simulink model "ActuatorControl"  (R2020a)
settings: Solver=FixedStepDiscrete  StartTime=0.0  StopTime=10.0  FixedStep=0.001  RelTol=1e-3  EnableMultiTasking=on
model workspace (MAT data in the model file):
  Ts : Simulink.Parameter (value not decoded)
symbols that are objects in the model workspace (value not decoded): Ts
undefined symbols (not defined in the file or in its folder): DiscIntNeverNeededParam
libraries: simulink x3

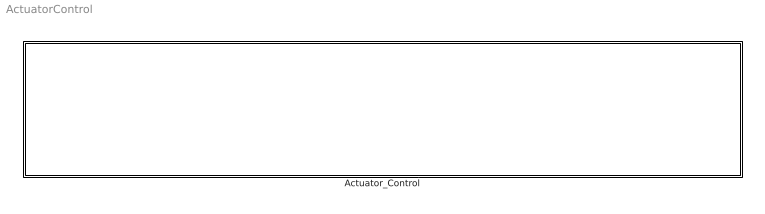
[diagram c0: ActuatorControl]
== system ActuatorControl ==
  Actuator_Control : Subsystem  TreatAsAtomicUnit=on

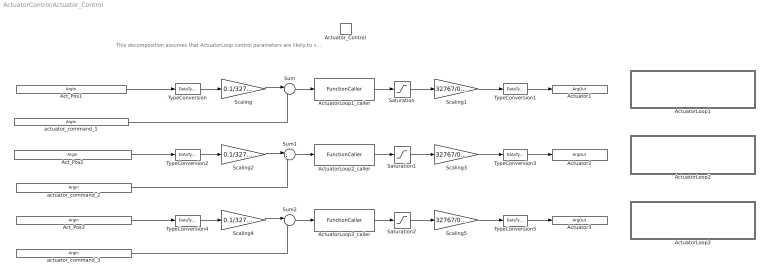
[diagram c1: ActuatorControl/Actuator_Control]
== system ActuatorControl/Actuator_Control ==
  note: This decomposition assumes that ActuatorLoop control parameters are likely to vary between actuators.
  Actuator_Control : TriggerPort  TriggerType=function-call  IsSimulinkFunction=on  FunctionName=Actuator_Control  FunctionVisibility=scoped  VariantControl=Variant  PortDimensions=1
  ActuatorLoop1 : Subsystem  TreatAsAtomicUnit=on
  ActuatorLoop1_caller : FunctionCaller  FunctionPrototype=Y = ActuatorLoop1(U)  InputArgumentSpecifications=double(1)  OutputArgumentSpecifications=double(1)
  ActuatorLoop2 : Subsystem  TreatAsAtomicUnit=on
  ActuatorLoop2_caller : FunctionCaller  FunctionPrototype=Y = ActuatorLoop2(U)  InputArgumentSpecifications=double(1)  OutputArgumentSpecifications=double(1)
  ActuatorLoop3 : Subsystem  TreatAsAtomicUnit=on
  ActuatorLoop3_caller : FunctionCaller  FunctionPrototype=Y = ActuatorLoop3(U)  InputArgumentSpecifications=double(1)  OutputArgumentSpecifications=double(1)
  Saturation : Saturate  UpperLimit=0.3  LowerLimit=-0.3
  Saturation1 : Saturate  UpperLimit=0.3  LowerLimit=-0.3
  Saturation2 : Saturate  UpperLimit=0.3  LowerLimit=-0.3
  Scaling : Gain  Gain=0.1/32767
  Scaling1 : Gain  Gain=32767/0.3  SaturateOnIntegerOverflow=on
  Scaling2 : Gain  Gain=0.1/32767
  Scaling3 : Gain  Gain=32767/0.3  SaturateOnIntegerOverflow=on
  Scaling4 : Gain  Gain=0.1/32767
  Scaling5 : Gain  Gain=32767/0.3  SaturateOnIntegerOverflow=on
  Sum : Sum  Inputs=|-+
  Sum1 : Sum  Inputs=|-+
  Sum2 : Sum  Inputs=|-+
  TypeConversion : DataTypeConversion  OutDataTypeStr=double
  TypeConversion1 : DataTypeConversion  OutDataTypeStr=int16
  TypeConversion2 : DataTypeConversion  OutDataTypeStr=double
  TypeConversion3 : DataTypeConversion  OutDataTypeStr=int16
  TypeConversion4 : DataTypeConversion  OutDataTypeStr=double
  TypeConversion5 : DataTypeConversion  OutDataTypeStr=int16
  Act_Pos1 : ArgIn  OutMin=-32768  OutMax=32767  OutDataTypeStr=int16  ArgumentName=Act_Pos1
  actuator_command_1 : ArgIn  Port=2  OutMin=-.1  OutMax=.1  ArgumentName=actuator_command_1
  Act_Pos2 : ArgIn  Port=3  OutMin=-32768  OutMax=32767  OutDataTypeStr=int16  ArgumentName=Act_Pos2
  actuator_command_2 : ArgIn  Port=4  OutMin=-.1  OutMax=.1  ArgumentName=actuator_command_2
  Act_Pos3 : ArgIn  Port=5  OutMin=-32768  OutMax=32767  OutDataTypeStr=int16  ArgumentName=Act_Pos3
  actuator_command_3 : ArgIn  Port=6  OutMin=-.1  OutMax=.1  ArgumentName=actuator_command_3
  Actuator1 : ArgOut  OutMin=-32768  OutMax=32767  OutDataTypeStr=int16  ArgumentName=Actuator1
  Actuator2 : ArgOut  Port=2  OutMin=-32768  OutMax=32767  OutDataTypeStr=int16  ArgumentName=Actuator2
  Actuator3 : ArgOut  Port=3  OutMin=-32768  OutMax=32767  OutDataTypeStr=int16  ArgumentName=Actuator3
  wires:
  ActuatorLoop1_caller/1 -> Saturation/1
  Saturation/1 -> Scaling1/1
  Scaling/1 -> Sum/1
  Scaling1/1 -> TypeConversion1/1
  Sum/1 -> ActuatorLoop1_caller/1
  actuator_command_1/1 -> Sum/2
  Act_Pos1/1 -> TypeConversion/1
  TypeConversion1/1 -> Actuator1/1
  TypeConversion/1 -> Scaling/1
  Scaling3/1 -> TypeConversion3/1
  TypeConversion2/1 -> Scaling2/1
  Sum1/1 -> ActuatorLoop2_caller/1
  TypeConversion3/1 -> Actuator2/1
  Scaling2/1 -> Sum1/1
  actuator_command_2/1 -> Sum1/2
  Saturation1/1 -> Scaling3/1
  Act_Pos2/1 -> TypeConversion2/1
  ActuatorLoop2_caller/1 -> Saturation1/1
  ActuatorLoop3_caller/1 -> Saturation2/1
  Scaling5/1 -> TypeConversion5/1
  actuator_command_3/1 -> Sum2/2
  Saturation2/1 -> Scaling5/1
  Act_Pos3/1 -> TypeConversion4/1
  Scaling4/1 -> Sum2/1
  TypeConversion5/1 -> Actuator3/1
  Sum2/1 -> ActuatorLoop3_caller/1
  TypeConversion4/1 -> Scaling4/1

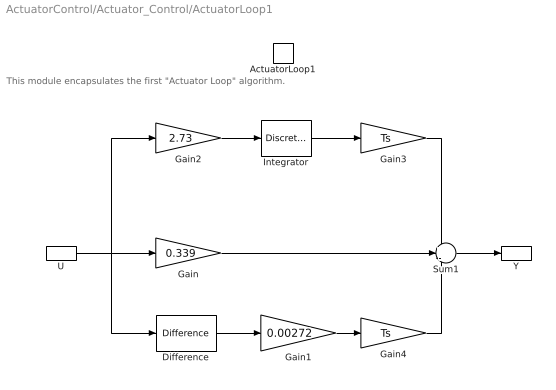
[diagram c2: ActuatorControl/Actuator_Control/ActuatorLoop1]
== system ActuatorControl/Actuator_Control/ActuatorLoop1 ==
  note: This module encapsulates the first "Actuator Loop" algorithm.
  ActuatorLoop1 : TriggerPort  TriggerType=function-call  IsSimulinkFunction=on  FunctionName=ActuatorLoop1  FunctionVisibility=scoped  VariantControl=Variant  PortDimensions=1
  Difference : simulink/Discrete/Difference  ICPrevInput=0.0  OutMin=[]  OutMax=[]  OutDataType=fixdt(1, 16)  OutScaling=2^-10  DoSatur=off
  Gain : Gain  Gain=0.339
  Gain1 : Gain  Gain=0.00272
  Gain2 : Gain  Gain=2.73
  Gain3 : Gain  Gain=Ts
  Gain4 : Gain  Gain=Ts
  Integrator : DiscreteIntegrator  IntegratorMethod=Accumulation: Forward Euler  SampleTime=-1  LimitOutput=on  UpperSaturationLimit=0.1  LowerSaturationLimit=-0.1  ICPrevOutput=DiscIntNeverNeededParam  ICPrevScaledInput=DiscIntNeverNeededParam
  Sum1 : Sum  Inputs=++-
  U : ArgIn  ArgumentName=U
  Y : ArgOut  ArgumentName=Y
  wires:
  Gain1/1 -> Gain4/1
  Sum1/1 -> Y/1
  U/1 -> Difference/1, Gain2/1, Gain/1
  Integrator/1 -> Gain3/1
  Gain2/1 -> Integrator/1
  Gain/1 -> Sum1/2
  Difference/1 -> Gain1/1
  Gain3/1 -> Sum1/1
  Gain4/1 -> Sum1/3

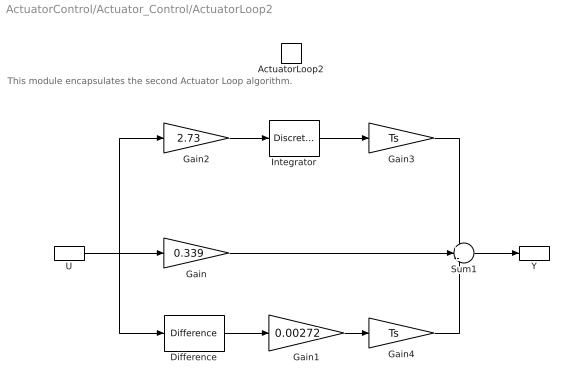
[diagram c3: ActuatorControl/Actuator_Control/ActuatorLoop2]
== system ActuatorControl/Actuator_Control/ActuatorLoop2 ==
  note: This module encapsulates the second Actuator Loop algorithm.
  ActuatorLoop2 : TriggerPort  TriggerType=function-call  IsSimulinkFunction=on  FunctionName=ActuatorLoop2  FunctionVisibility=scoped  VariantControl=Variant  PortDimensions=1
  Difference : simulink/Discrete/Difference  ICPrevInput=0.0  OutMin=[]  OutMax=[]  OutDataType=fixdt(1, 16)  OutScaling=2^-10  DoSatur=off
  Gain : Gain  Gain=0.339
  Gain1 : Gain  Gain=0.00272
  Gain2 : Gain  Gain=2.73
  Gain3 : Gain  Gain=Ts
  Gain4 : Gain  Gain=Ts
  Integrator : DiscreteIntegrator  IntegratorMethod=Accumulation: Forward Euler  SampleTime=-1  LimitOutput=on  UpperSaturationLimit=0.1  LowerSaturationLimit=-0.1  ICPrevOutput=DiscIntNeverNeededParam  ICPrevScaledInput=DiscIntNeverNeededParam
  Sum1 : Sum  Inputs=++-
  U : ArgIn  ArgumentName=U
  Y : ArgOut  ArgumentName=Y
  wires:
  Difference/1 -> Gain1/1
  Gain/1 -> Sum1/2
  Gain2/1 -> Integrator/1
  Integrator/1 -> Gain3/1
  U/1 -> Gain/1, Gain2/1, Difference/1
  Sum1/1 -> Y/1
  Gain1/1 -> Gain4/1
  Gain3/1 -> Sum1/1
  Gain4/1 -> Sum1/3

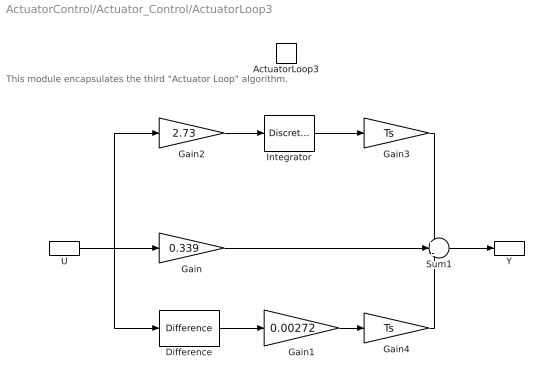
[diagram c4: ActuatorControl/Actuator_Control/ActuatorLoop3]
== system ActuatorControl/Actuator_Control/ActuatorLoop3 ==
  note: This module encapsulates the third "Actuator Loop" algorithm.
  ActuatorLoop3 : TriggerPort  TriggerType=function-call  IsSimulinkFunction=on  FunctionName=ActuatorLoop3  FunctionVisibility=scoped  VariantControl=Variant  PortDimensions=1
  Difference : simulink/Discrete/Difference  ICPrevInput=0.0  OutMin=[]  OutMax=[]  OutDataType=fixdt(1, 16)  OutScaling=2^-10  DoSatur=off
  Gain : Gain  Gain=0.339
  Gain1 : Gain  Gain=0.00272
  Gain2 : Gain  Gain=2.73
  Gain3 : Gain  Gain=Ts
  Gain4 : Gain  Gain=Ts
  Integrator : DiscreteIntegrator  IntegratorMethod=Accumulation: Forward Euler  SampleTime=-1  LimitOutput=on  UpperSaturationLimit=0.1  LowerSaturationLimit=-0.1  ICPrevOutput=DiscIntNeverNeededParam  ICPrevScaledInput=DiscIntNeverNeededParam
  Sum1 : Sum  Inputs=++-
  U : ArgIn  ArgumentName=U
  Y : ArgOut  ArgumentName=Y
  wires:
  Gain1/1 -> Gain4/1
  Sum1/1 -> Y/1
  U/1 -> Difference/1, Gain2/1, Gain/1
  Integrator/1 -> Gain3/1
  Gain2/1 -> Integrator/1
  Gain/1 -> Sum1/2
  Difference/1 -> Gain1/1
  Gain3/1 -> Sum1/1
  Gain4/1 -> Sum1/3
